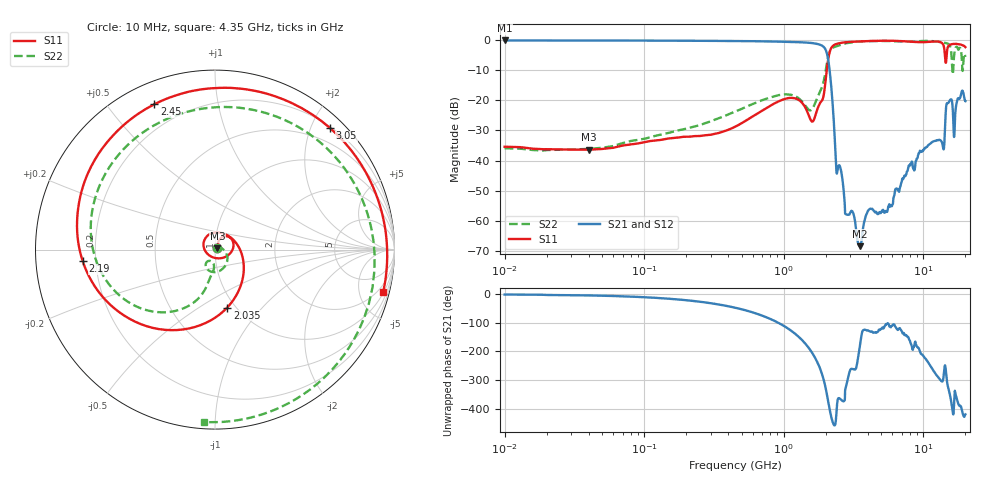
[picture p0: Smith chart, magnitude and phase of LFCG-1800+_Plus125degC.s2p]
! Mini-Circuits
! S2P DATA File Format
! Type: LOW PASS FILTER
! Model: LFCG-1800+
! All S Parameters are in dB deg format
! TEST CONDITIONS: INPUT POWER = 0 dBm @ Temperature = +125deg C
!S2P File: Measurements: S11, S21, S12, S22:
# Hz S  dB  R 50
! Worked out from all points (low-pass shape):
!   718 points, 10 MHz to 20 GHz, reference 50 ohm
!   highest |S21| = -0.14 dB at 10 MHz (marker M1); lowest = -68.4 dB at 3.5 GHz (marker M2)
!   |S21| within 3 dB of the highest: start of sweep to 1.991 GHz
!   lowest |S11| = -36.4 dB at 40 MHz (marker M3), VSWR 1.03, Z = 51.4 + j0.695 ohm
!   |S11| at or under -10 dB: start of sweep to 2.031 GHz
!   |S22| runs from -36.6 to -0.3 dB; largest |S21 - S12| = 0.00058
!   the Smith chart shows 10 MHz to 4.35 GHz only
!   S11 on the Smith chart (normalised r, x): 10 MHz: 1.03, +0.02; 2.035 GHz: 0.92, -0.66; 2.19 GHz: 0.15, -0.04; 2.45 GHz: 0.09, +0.66; 3.05 GHz: 0.22, +2.31; 4.35 GHz: 1.11, -7.89
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1e7  -35.39 42.4  -0.14 -1.6  -0.14 -1.6  -35.90 40.6
4e7  -36.38 26.5  -0.15 -4.6  -0.15 -4.6  -36.11 25.9
1.3e8  -33.16 37.6  -0.20 -14.0  -0.20 -14.0  -31.43 25.4
4.5e8  -28.69 62.3  -0.32 -47.7  -0.32 -47.7  -23.70 -17.3
1.01e9  -19.58 41.9  -0.58 -112.2  -0.58 -112.2  -18.02 -89.5
1.59e9  -27.03 -108.4  -0.99 156.3  -1.00 156.3  -22.99 -102.3
1.855e9  -20.40 88.5  -1.73 88.8  -1.73 88.8  -16.20 -99.5
2.035e9  -9.63 -78.1  -4.38 10.7  -4.38 10.7  -7.81 -122.9
2.19e9  -2.62 -174.9  -15.67 -69.5  -15.68 -69.5  -2.95 165.5
2.45e9  -1.14 112.7  -42.13 -5.0  -42.13 -4.9  -1.87 75.1
3.05e9  -0.61 46.5  -56.64 99.3  -56.65 99.3  -0.78 -24.4
3.5e9  -0.46 19.0  -68.37 175.0  -68.36 175.8  -0.49 -58.8
4.35e9  -0.30 -14.2  -56.27 -134.3  -56.27 -134.5  -0.33 -93.6
5.65e9  -0.23 -42.4  -54.93 -105.2  -54.93 -105.3  -0.34 -122.9
9.05e9  -0.67 -83.2  -39.17 174.6  -39.17 174.7  -0.41 174.6
1.205e10  -0.48 -116.6  -33.47 86.4  -33.47 86.4  -0.43 115.0
1.395e10  -1.81 -171.0  -36.25 71.7  -36.25 71.7  -0.83 79.6
1.5e10  -2.23 -177.9  -20.93 36.5  -20.94 36.5  -1.22 59.4
1.615e10  -1.32 137.6  -21.53 -45.3  -21.54 -45.4  -10.80 -67.6
1.66e10  -1.32 128.8  -32.16 -17.8  -32.18 -17.7  -5.16 143.0
1.72e10  -1.24 122.4  -21.48 1.6  -21.48 1.7  -2.26 106.0
2e10  -2.35 106.9  -20.29 -60.0  -20.33 -59.9  -5.60 102.7
